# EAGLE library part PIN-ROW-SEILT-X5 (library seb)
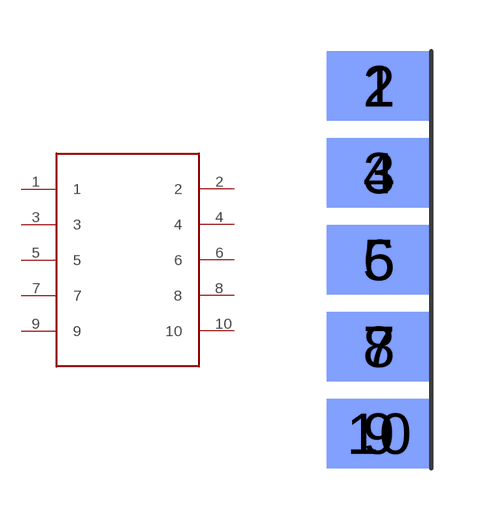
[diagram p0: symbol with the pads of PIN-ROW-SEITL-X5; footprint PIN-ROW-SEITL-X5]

Designator prefix X

## PIN-ROW-SEILT-X5  [PIN-ROW-SEITL-X5]
1  1
2  2
3  3
4  4
5  5
6  6
7  7
8  8
9  9
10  10

## Footprint PIN-ROW-SEITL-X5 (pad centres in mm)
smd 3.048 x 2.032: 1 1.524,11.176; 3 1.524,8.636; 5 1.524,6.096; 7 1.524,3.556; 9 1.524,1.016
smd 3.048 x 2.032 bottom: 2 1.524,11.176; 4 1.524,8.636; 6 1.524,6.096; 8 1.524,3.556; 10 1.524,1.016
